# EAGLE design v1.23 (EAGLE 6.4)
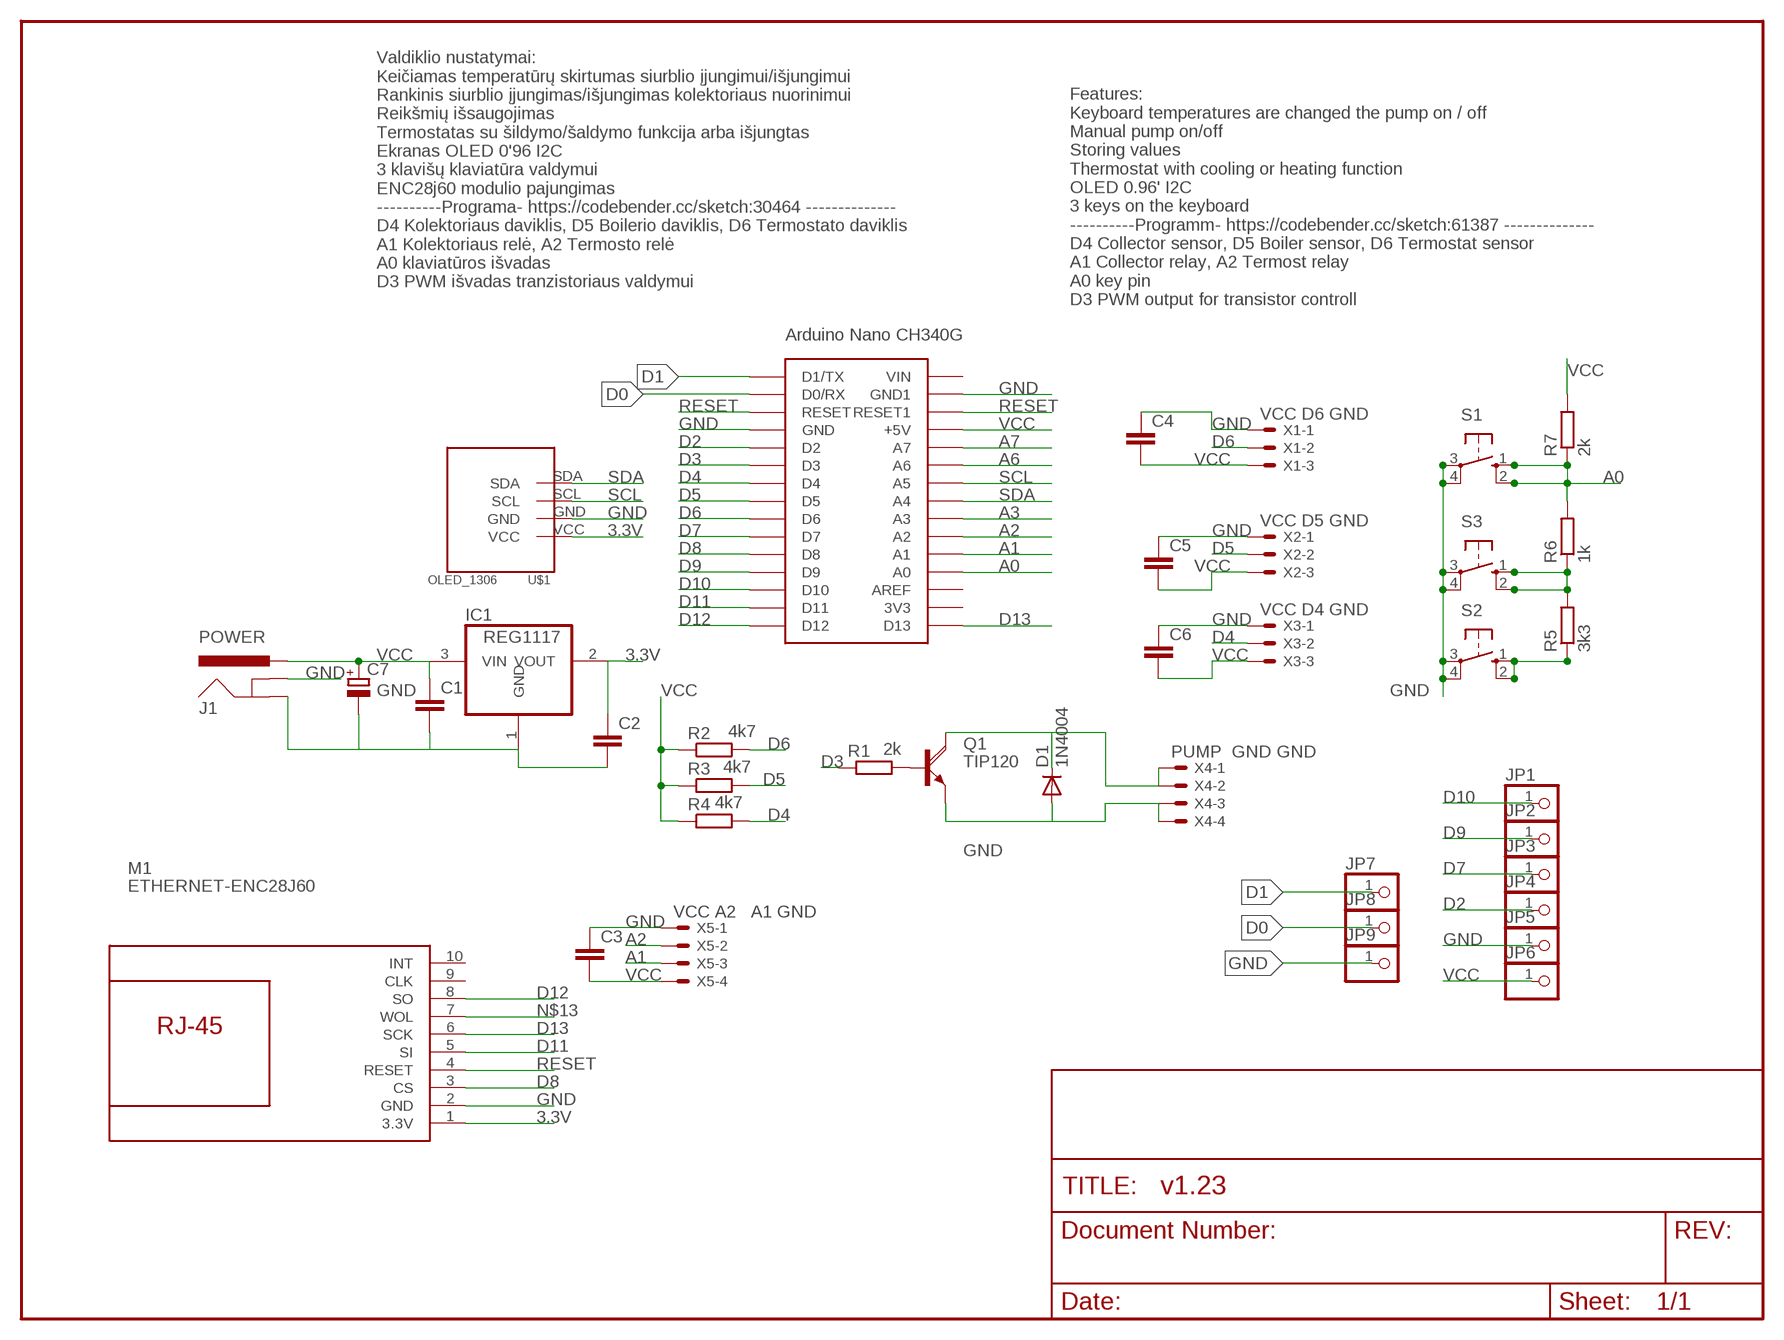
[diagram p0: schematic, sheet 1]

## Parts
ARDUINONANOCH340G  ARDUINONANO  [PDIP-32]
C1  C2,5-3  [C2.5-3]
C2  C2,5-3  [C2.5-3]
C3  C2,5-3  [C2.5-3]
C4  C2,5-3  [C2.5-3]
C5  C2,5-3  [C2.5-3]
C6  C2,5-3  [C2.5-3]
C7  CPOL-EUE2,5-6E  [E2,5-6E]
D1  1N4004  [DO41-10]
IC1  REG1117  [SOT223]
J1  POWER  POWER_JACKPTH_LOCK  [POWER_JACK_PTH_LOCK]
JP1  PINHD-1X1  [1X01]
JP2  PINHD-1X1  [1X01]
JP3  PINHD-1X1  [1X01]
JP4  PINHD-1X1  [1X01]
JP5  PINHD-1X1  [1X01]
JP6  PINHD-1X1  [1X01]
JP7  PINHD-1X1  [1X01]
JP8  PINHD-1X1  [1X01]
JP9  PINHD-1X1  [1X01]
M1  ETHERNET-ENC28J60  [ETHERNET-ENC28J60]
Q1  TIP120  [TO220AH]
R1  2k  R-EU_0207/10  [0207/10]
R2  4k7  R-EU_0207/10  [0207/10]
R3  4k7  R-EU_0207/10  [0207/10]
R4  4k7  R-EU_0207/10  [0207/10]
R5  3k3  R-EU_0207/10  [0207/10]
R6  1k  R-EU_0207/10  [0207/10]
R7  2k  R-EU_0207/10  [0207/10]
S1  10-XX  [B3F-10XX]
S2  10-XX  [B3F-10XX]
S3  10-XX  [B3F-10XX]
U$1  OLED_1306  [OLED_1306]
X1  VCC D6 GND  22-23-2031  [22-23-2031]
X2  VCC D5 GND  22-23-2031  [22-23-2031]
X3  VCC D4 GND  22-23-2031  [22-23-2031]
X4  PUMP GND GND  22-23-2041  [22-23-2041]
X5  VCC A2 A1 GND  22-23-2041  [22-23-2041]

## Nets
3.3V: C2.1 IC1.2(VOUT) M1.1(3.3V) U$1.VCC
A0: ARDUINONANOCH340G.A0 R6.2 R7.1 S1.1(S) S1.2(S1)
A1: ARDUINONANOCH340G.A1 X5.3
A2: ARDUINONANOCH340G.A2 X5.2
A3: ARDUINONANOCH340G.A3
A6: ARDUINONANOCH340G.A6
A7: ARDUINONANOCH340G.A7
D0: ARDUINONANOCH340G.D0/RX JP8.1
D1: ARDUINONANOCH340G.D1/TX JP7.1
D2: ARDUINONANOCH340G.D2 JP4.1
D3: ARDUINONANOCH340G.D3 R1.1
D4: ARDUINONANOCH340G.D4 R4.2 X3.2
D5: ARDUINONANOCH340G.D5 R3.2 X2.2
D6: ARDUINONANOCH340G.D6 R2.2 X1.2
D7: ARDUINONANOCH340G.D7 JP3.1
D8: ARDUINONANOCH340G.D8 M1.3(CS)
D9: ARDUINONANOCH340G.D9 JP2.1
D10: ARDUINONANOCH340G.D10 JP1.1
D11: ARDUINONANOCH340G.D11 M1.5(SI)
D12: ARDUINONANOCH340G.D12 M1.8(SO)
D13: ARDUINONANOCH340G.D13 M1.6(SCK)
GND [vcc]: ARDUINONANOCH340G.GND ARDUINONANOCH340G.GND1 C1.2 C2.2 C3.1 C4.1 C5.1 C6.1 C7.- D1.A IC1.1(GND) J1.GND J1.GNDBREAK JP5.1 JP9.1 M1.2(GND) Q1.E S1.3(P) S1.4(P1) S2.3(P) S2.4(P1) S3.3(P) S3.4(P1) U$1.GND X1.1 X2.1 X3.1 X4.3 X4.4 X5.1
N$1: Q1.B R1.2
N$2: D1.C Q1.C X4.1 X4.2
N$5: R5.1 S2.1(S) S2.2(S1)
N$6: R5.2 R6.1 S3.1(S) S3.2(S1)
N$13: M1.7(WOL)
RESET: ARDUINONANOCH340G.RESET ARDUINONANOCH340G.RESET1 M1.4(RESET)
SCL: ARDUINONANOCH340G.A5 U$1.SCL
SDA: ARDUINONANOCH340G.A4 U$1.SDA
VCC: ARDUINONANOCH340G.+5V C1.1 C3.2 C4.2 C5.2 C6.2 C7.+ IC1.3(VIN) J1.PWR JP6.1 R2.1 R3.1 R4.1 R7.2 X1.3 X2.3 X3.3 X5.4
Unconnected: ARDUINONANOCH340G.3V3 ARDUINONANOCH340G.AREF ARDUINONANOCH340G.VIN M1.9(CLK) M1.10(INT)

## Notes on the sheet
- Valdiklio nustatymai:
  Keičiamas temperatūrų skirtumas siurblio įjungimui/išjungimui
  Rankinis siurblio įjungimas/išjungimas kolektoriaus nuorinimui
  Reikšmių išsaugojimas
  Termostatas su šildymo/šaldymo funkcija arba išjungtas
  Ekranas OLED 0'96 I2C
  3 klavišų klaviatūra valdymui
  ENC28j60 modulio pajungimas
  ----------Programa- https://codebender.cc/sketch:30464 --------------
  D4 Kolektoriaus daviklis, D5 Boilerio daviklis, D6 Termostato daviklis
  A1 Kolektoriaus relė, A2 Termosto relė
  A0 klaviatūros išvadas 
  D3 PWM išvadas tranzistoriaus valdymui
- Features:
  Keyboard temperatures are changed the pump on / off
  Manual pump on/off
  Storing values
  Thermostat with cooling or heating function
  OLED 0.96' I2C
  3 keys on the keyboard
  ----------Programm- https://codebender.cc/sketch:61387 --------------
  D4 Collector sensor, D5 Boiler sensor, D6 Termostat sensor
  A1 Collector relay, A2 Termost relay
  A0 key pin 
  D3 PWM output for transistor controll
- Arduino Nano CH340G

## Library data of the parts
ARDUINONANOCH340G = rocketfarm:ARDUINONANO
C1-C6 = capacitor-wima:C: CAPACITOR
C7 = resistor:CPOL-EU: POLARIZED CAPACITOR, European symbol
D1 = diode:1N4004: DIODE
IC1 = burr-brown:REG1117: 800mA and 1A Low Dropout (LDO) Positive Regulator 1.8V, 2.5V, 2.85V, 3.3V, 5V, and Adj; MPN: REG1117; OC_FARNELL: 1097566; OC_NEWARK: 14P6981
J1 = SparkFun-Connectors:POWER_JACK: Power Jack This is the standard 5.5mm barrel jack for power. The PTH is the most common, proven, reliable, footprint. The Slot footprint only works if the mill layer is transmitted to the PCB fab house so be warned. Spark Fun Electronics SKU : PRT-00119 SMT: CONN-08106 Mating wall wart : TOL-00298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
JP1-JP9 = pinhead:PINHD-1X1: PIN HEADER
M1 = diy-modules:ETHERNET-ENC28J60: Ethernet Module based on ENC28J60 chip
Q1 = transistor-power:TIP120: NPN DARLINGTON TRANSISTOR
R1-R7 = resistor:R-EU_: RESISTOR, European symbol
S1-S3 = switch-omron:10-XX: OMRON SWITCH; MPN: B3F-1000; OC_FARNELL: 176432; OC_NEWARK: 36M3542
U$1 = tft_1.8:OLED_1306
X1-X3 = con-molex:22-23-2031: .100" (2.54mm) Center Header - 3 Pin; MF: MOLEX; MPN: 22-23-2031; OC_FARNELL: 1462950; OC_NEWARK: 30C0862
X4 X5 = con-molex:22-23-2041: .100" (2.54mm) Center Header - 4 Pin; MF: MOLEX; MPN: 22-23-2041; OC_FARNELL: 1462920; OC_NEWARK: 38C0355

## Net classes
0 default: width 0.3 mm
1 vcc: width 0.4 mm
2 gnd: width 0.5 mm

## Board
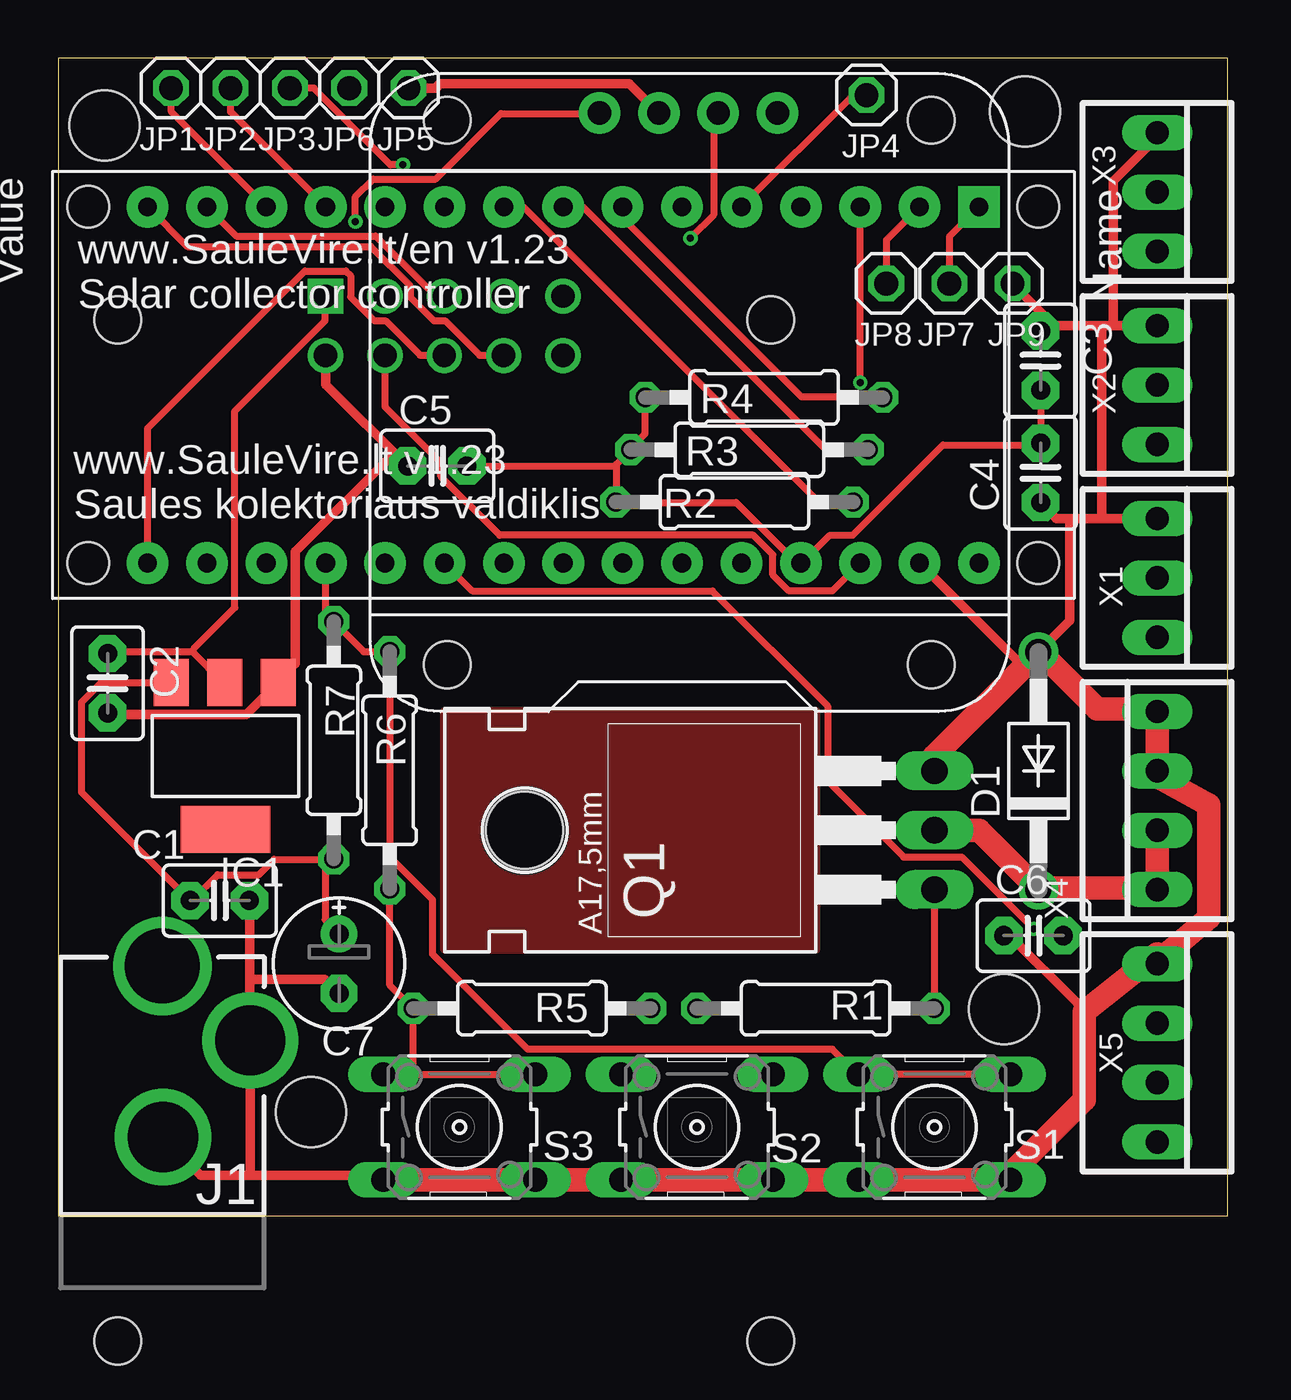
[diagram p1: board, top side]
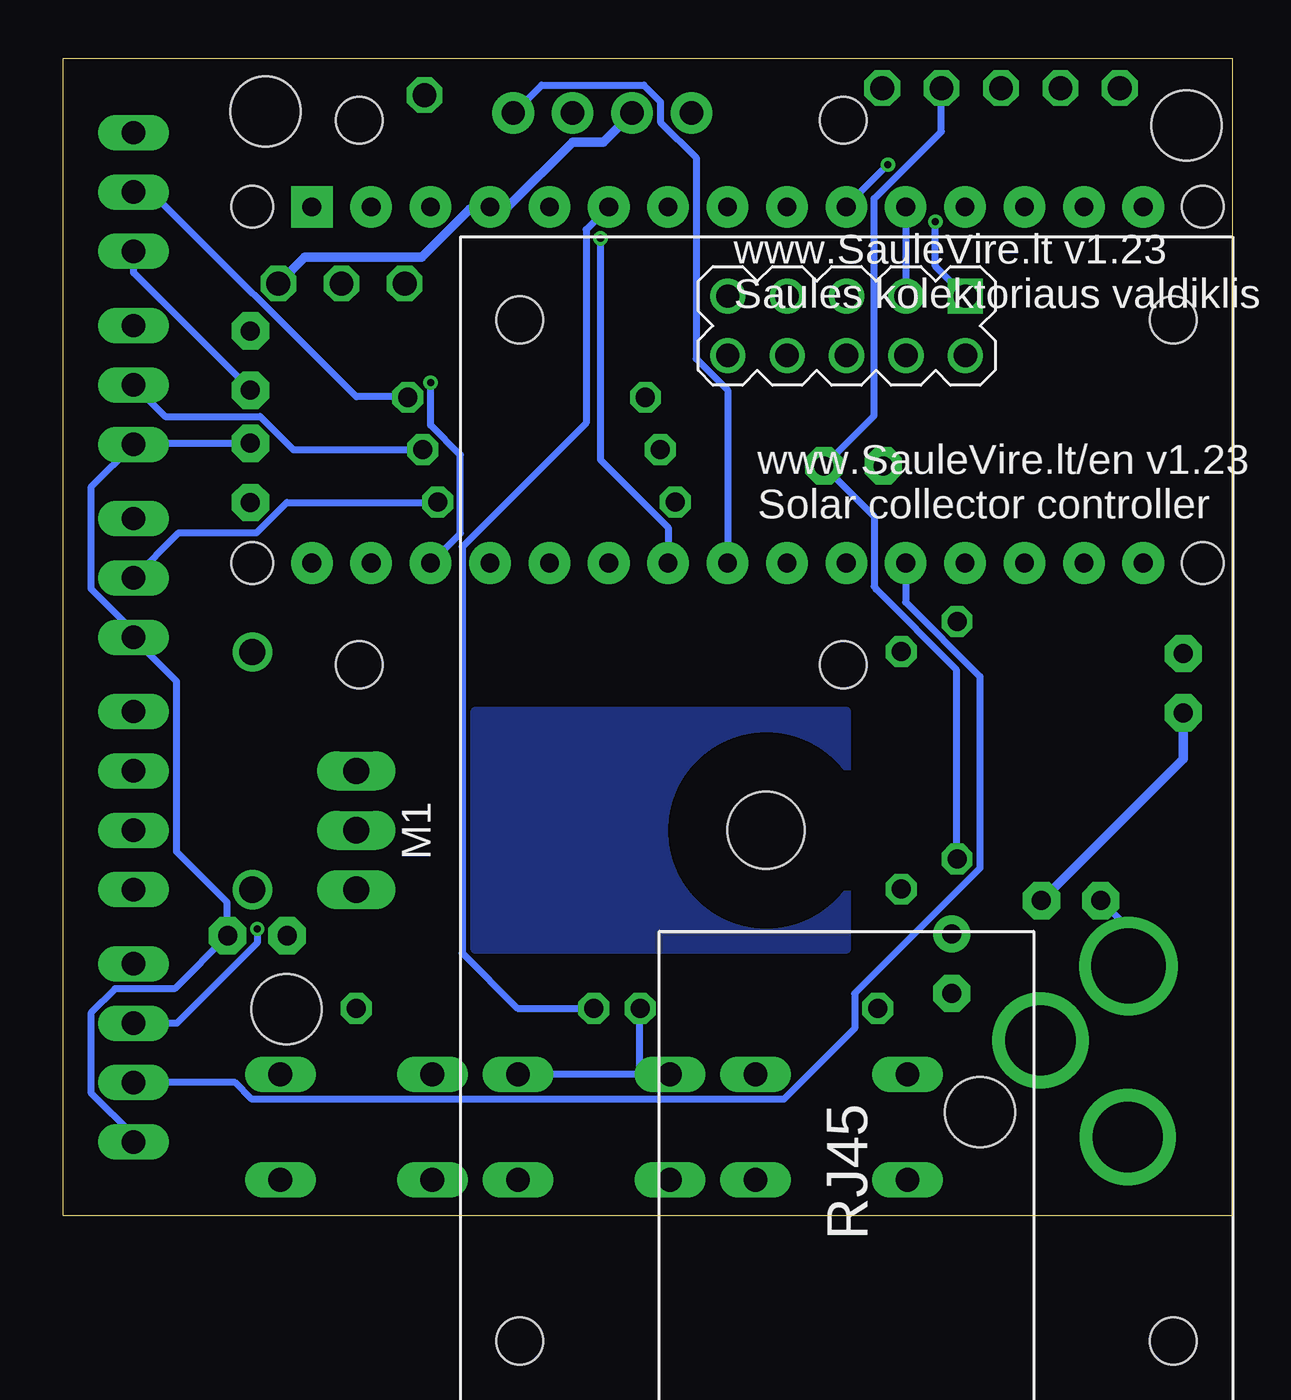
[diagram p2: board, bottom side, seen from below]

Size 50 x 49.51 mm. Coordinates in mm from the lower left corner, seen from the top.
Outline: 0,49.51 0,0 50,0 50,49.51 0,49.51
Copper layers (1*16): Top 0.035mm / dielectric 1.5mm / Bottom 0.035mm
Design rules "ITEADstudio_DRC": minimum track width 6mil, minimum drill 12mil, track to track 6mil, track to pad 6mil, pad to pad 6mil, via to via 6mil, smd to smd 0mil, copper to edge 10mil, drill to drill 10mil, minimum pad ring 10mil, minimum via ring 6mil, stop-mask expansion 2mil, vias tented up to drill 100mil, thermal gap 10mil
Holes 3 mm at 1.97,46.64 10.79,4.43 40.45,8.84 41.34,47.24

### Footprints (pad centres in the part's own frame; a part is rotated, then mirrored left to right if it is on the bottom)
PDIP-32 = drill 0.8 pad 1.778: 3V3 15.24,-35.56; +5V 15.24,-10.16; A0 15.24,-30.48; A1 15.24,-27.94; A2 15.24,-25.4; A3 15.24,-22.86; A4 15.24,-20.32; A5 15.24,-17.78; A6 15.24,-15.24; A7 15.24,-12.7; AREF 15.24,-33.02; D0/RX 0,-5.08; D2 0,-12.7; D3 0,-15.24; D4 0,-17.78; D5 0,-20.32; D6 0,-22.86; D7 0,-25.4; D8 0,-27.94; D9 0,-30.48; D10 0,-33.02; D11 0,-35.56; D12 0,-38.1; D13 15.24,-38.1; GND 0,-10.16; GND1 15.24,-5.08; RESET 0,-7.62; RESET1 15.24,-7.62; VIN 15.24,-2.54 | drill 0.8 pad 1.778 square: D1/TX 0,-2.54 | hole 1.778: 0,0; 0,-40.64; 15.24,-40.64; 15.24,0
C2.5-3 = drill 0.813 pad 1.6 octagon: 1 -1.27,0; 2 1.27,0
E2,5-6E = drill 0.813 pad 1.575: + -1.27,0 | drill 0.813 pad 1.575 octagon: - 1.27,0
DO41-10 = drill 1.118: A 5.08,0; C -5.08,0
SOT223 = smd 1.499 x 2.007: 1 -2.261,-3.15; 2 0.025,-3.15; 3 2.311,-3.15 | smd 3.81 x 2.007: 4 0,3.15
POWER_JACK_PTH_LOCK = drill 2.997 pad 4.115: GND 0.025,6.557; GNDBREAK 3.762,10.7 | drill 3.2 pad 4.115: PWR 0,13.878
1X01 = drill 1.016 octagon: 1 0,0
ETHERNET-ENC28J60 = drill 1 square: 1 22.86,-5.08 | drill 1: 2 20.32,-5.08; 3 22.86,-2.54; 4 20.32,-2.54; 5 22.86,0; 6 20.32,0; 7 22.86,2.54; 8 20.32,2.54; 9 22.86,5.08; 10 20.32,5.08 | hole 2: -21.844,13.97; 21.844,13.97; -21.844,-13.97; 21.844,-13.97
TO220AH = drill 1.118 long: B -2.54,-6.35; C 0,-6.35; E 2.54,-6.35 | hole 3.302: 0,11.176
0207/10 = drill 0.813 octagon: 1 -5.08,0; 2 5.08,0
B3F-10XX = drill 1.016 long: 1 -3.251,2.261; 2 3.251,2.261; 3 -3.251,-2.261; 4 3.251,-2.261
OLED_1306 = drill 1 pad 1.778: GND -0.36,11.63; SCL 2.18,11.63; SDA 4.72,11.63; VCC -2.9,11.63 | hole 2: -9.4,-11.97; 11.3,-11.97; 11.3,11.33; -9.4,11.33
22-23-2031 = drill 1 long: 1 -2.54,0; 2 0,0; 3 2.54,0
22-23-2041 = drill 1 long: 1 -3.81,0; 2 -1.27,0; 3 1.27,0; 4 3.81,0

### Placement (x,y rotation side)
ARDUINONANOCH340G  41.91,43.16 270 top
C1  6.9,13.48 0 top
C2  2.1,22.78 270 top
C3  42,36.58 270 top
C4  42,31.78 90 top
C5  16.2,32.08 0 top
C6  41.7,11.98 0 top
C7  12,10.78 270 top
D1  41.91,19.03 90 top
IC1  7.14,19.66 180 top
J1  4.45,-3.19 0 top
JP1  4.82,48.24 0 top
JP2  7.36,48.24 0 top
JP3  9.89,48.24 0 top
JP4  34.55,47.94 0 top
JP5  14.97,48.24 0 top
JP6  12.44,48.24 0 top
JP7  38.1,39.88 0 top
JP8  35.4,39.88 0 top
JP9  40.8,39.88 0 top
M1  16.5,16.48 90 bottom
Q1  31.11,16.49 90 top
R1  32.38,8.87 0 top
R2  28.91,30.53 0 top
R3  29.55,32.77 0 top
R4  30.18,35.01 0 top
R5  20.25,8.87 180 top
R6  14.16,19.05 90 top
R7  11.78,20.34 270 top
S1  37.47,3.79 0 top
S2  27.3,3.79 0 top
S3  17.14,3.79 0 top
U$1  26.04,35.54 0 top
X1  46.99,27.29 270 top
X2  46.99,35.54 270 top
X3  46.99,43.79 270 top
X4  46.99,17.76 90 top
X5  46.99,6.97 270 top

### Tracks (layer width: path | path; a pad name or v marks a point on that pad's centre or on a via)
3.3V  (via drill 0.3)
  Top 0.3: IC1.2 7.04,22.82 5.71,24.14 | 5.71,24.14 2.18,24.14 C2.1 | M1.1 11.4,39.32 11.4,38.28 7.54,34.42 7.54,26.02 5.79,24.26 5.71,24.14 | v12.7,42.52 12.7,43.59 13.46,44.35 16.13,44.35 18.92,47.15 23.11,47.15 U$1.VCC
  Bottom 0.3: v12.7,42.52 12.7,40.62 M1.1
A0
  Top 0.3: S1.2 S1.1 34.09,6.13 33.1,7.12 20.07,7.12 16,11.18 16,13.52 14.2,15.32 14.2,23.98 R6.2 14.15,24.14 13.06,24.14 11.89,25.3 R7.1 11.71,25.56 11.43,25.84 ARDUINONANOCH340G.A0
A1
  Bottom 0.3: X5.3 42.65,5.7 41.94,4.98 19.18,4.98 16.15,8.01 16.15,9.51 10.79,14.86 10.79,23.07 13.97,26.24 ARDUINONANOCH340G.A1
A2  (via drill 0.3)
  Top 0.3: v41.71,12.27 38.63,15.35 36.14,15.35 32.89,18.6 32.89,21.8 27.96,26.73 17.7,26.73 ARDUINONANOCH340G.A2
  Bottom 0.3: X5.2 45.14,8.24 41.71,11.66 v41.71,12.27
D0
  Top 0.3: ARDUINONANOCH340G.D0/RX 35.41,41.74 JP8.1
D1
  Top 0.3: JP7.1 38.1,41.89 ARDUINONANOCH340G.D1/TX
D2
  Top 0.3: ARDUINONANOCH340G.D2 33.98,47.93 JP4.1
D3
  Bottom 0.3: R1.1 30.58,8.87 32.94,11.23 32.94,28.61 27.64,33.91 27.64,42.2 ARDUINONANOCH340G.D3
D4
  Top 0.3: ARDUINONANOCH340G.D4 24.13,42.68 31.77,35.03 35.26,35.03 R4.2
  Bottom 0.3: X3.2 46.23,43.79 37.47,35.03 35.28,35.03 R4.2
D5
  Top 0.3: ARDUINONANOCH340G.D5 22.43,43.16 32.82,32.77 R3.2
  Bottom 0.3: X2.2 45.64,34.19 41.58,34.19 40.16,32.77 34.65,32.77 R3.2
D6
  Top 0.3: ARDUINONANOCH340G.D6 19.89,43.16 32.51,30.54 R2.2
  Bottom 0.3: X1.2 45.06,29.21 41.73,29.21 40.44,30.51 34.01,30.51 R2.2
D7  (via drill 0.3)
  Top 0.3: JP3.1 10.92,48.24 14.2,44.96 v14.73,44.96
  Bottom 0.3: v14.73,44.96 16.51,43.18 ARDUINONANOCH340G.D7
D8
  Bottom 0.3: ARDUINONANOCH340G.D8 M1.3
D9
  Top 0.3: ARDUINONANOCH340G.D9 7.37,47.22 JP2.1
D10
  Top 0.3: ARDUINONANOCH340G.D10 4.83,47.22 JP1.1
D11
  Top 0.3: ARDUINONANOCH340G.D11 7.59,41.91 13.56,41.91 16.13,39.35 16.48,39.35 M1.5
D12
  Top 0.3: ARDUINONANOCH340G.D12 5.51,41.46 13.36,41.46 15.04,39.78 15.04,39.3 16.05,38.28 16.54,38.28 18.01,36.81 19.02,36.81 M1.8
D13
  Top 0.3: ARDUINONANOCH340G.D13 3.81,33.69 10.54,40.42 12.29,40.42 12.5,40.21 12.5,39.3 13.51,38.28 13.99,38.28 15.47,36.81 16.48,36.81 M1.6
GND
  Top 0.4: 46.99,11.21 X5.1 47.09,10.95 | 40.92,2.01 S1.4 | D1.A 41.26,23.46 40.95,23.8 ARDUINONANOCH340G.GND1 | 46.81,21.67 X4.4 | 42.09,24.01 D1.A | 42.22,24.16 D1.A | 47.09,18.73 47.09,18.85 X4.3 | 8.2,1.73 6.1,1.73 J1.GND | 8.2,1.73 13.41,1.73 S3.3 | 8.2,1.73 8.2,7.3 J1.GNDBREAK 8.18,7.7 8.18,10.12 | JP5.1 16.13,48.24 16.31,48.42 24.41,48.42 25.65,47.17 U$1.GND | 44.63,38.08 42.24,38.08 42.01,37.85 C3.1 42.42,38.26 40.82,39.86 JP9.1 | 44.63,38.08 45.11,38.08 | 45.11,38.08 X2.1 | X3.1 46.99,46.13 45.11,44.25 45.11,38.08 | M1.2 11.43,36.78 11.43,35.56 14.91,32.09 C5.1 14.22,32.49 10.13,28.4 10.13,23.63 9.5,22.99 IC1.1 9.4,22.82 8.03,21.44 2.16,21.44 2.11,21.49 C2.2 | 43.26,29.82 42.67,29.82 42.01,30.48 C4.1 | 43.26,29.82 44.63,29.82 | 44.63,29.82 X1.1 | 8.18,10.12 8.18,13.47 C1.2 | C6.1 40.69,11.97 43.56,9.1 43.87,8.72 | 43.26,29.82 43.26,25.46 D1.A | 44.63,29.82 44.63,38.08 | 8.18,10.12 11.38,10.12 C7.-
  Top 1: S3.3 S3.4 S2.3 S2.4 S1.3 S1.4 | 46.99,11.21 43.87,8.72 43.87,4.96 40.92,2.01 | X4.4 X4.3 | Q1.E 37.47,19.66 41.26,23.46 | 46.81,21.67 44.42,21.67 42.09,24.01 | 47.09,18.73 49.2,17.58 49.2,12.73 47.09,10.95
  Bottom 0.4: U$1.GND 25.68,47.15 26.9,45.93 28.22,45.93 30.99,43.16 ARDUINONANOCH340G.GND 31.93,43.06 32.61,43.06 34.67,41 39.67,41 JP9.1 | C2.2 2.11,21.49 2.11,19.54 8.15,13.49 C1.2
N$1
  Top 0.3: Q1.B R1.2
N$2
  Top 0.3: 46.86,14.03 X4.1 | 42.04,14.03 D1.C
  Top 1: X4.2 X4.1 | Q1.C 39.37,16.49 D1.C | 42.04,14.03 46.86,14.03
N$3
  pour Bottom: 16.51,21.57 32.38,21.57 32.38,11.41 16.51,11.41
N$4
  pour Top: 16.51,21.57 32.38,21.57 32.38,11.41 16.51,11.41
N$5
  Bottom 0.3: S2.1 S2.2 | 24.13,6.18 S2.1 | R5.1 25.35,8.87 25.35,6.18 S2.1
N$6
  Top 0.3: S3.2 S3.1 15.16,6.18 15.16,8.74 R5.2 14.17,9.86 14.17,13.95 R6.1
RESET  (via drill 0.3)
  Top 0.3: ARDUINONANOCH340G.RESET1 33.1,26.73 31.24,26.73 30.56,27.41 30.56,28.28 29.72,29.11 18.87,29.11 16.36,31.63 16.36,32.21 13.97,34.6 13.97,36.78 M1.4 | v34.29,35.64 ARDUINONANOCH340G.RESET
  Bottom 0.3: v34.29,35.64 34.29,33.81 33.02,32.54 33.02,29.19 ARDUINONANOCH340G.RESET1
SCL  (via drill 0.3)
  Top 0.3: v27.03,41.81 28.02,42.8 28.02,46.97 28.19,47.15 U$1.SCL
  Bottom 0.3: ARDUINONANOCH340G.A5 24.13,29.44 27.03,32.34 v27.03,41.81
SDA
  Bottom 0.3: ARDUINONANOCH340G.A4 21.59,35.31 22.94,36.66 22.94,45.27 24.46,46.79 24.46,47.66 25.17,48.37 29.54,48.37 30.73,47.17 U$1.SDA
VCC
  Top 0.3: C3.2 42.01,35.29 42.01,33.05 C4.2 41.86,32.97 37.82,32.97 33.96,29.11 32.99,29.11 31.88,28 ARDUINONANOCH340G.+5V 31.57,27.92 28.98,30.51 24,30.51 R2.1 23.85,30.54 23.85,32.06 | IC1.3 1.83,22.82 0.99,21.98 0.99,18.12 5.61,13.49 C1.1 5.77,13.54 6.81,14.59 8.56,14.59 9.22,15.25 11.76,15.25 R7.2 11.4,15.12 11.4,12.66 C7.+ | 23.85,32.06 23.85,32.14 24.46,32.75 R3.1 24.54,32.9 25.09,33.46 R4.1 | 23.85,32.06 17.48,32.06 C5.2
  Bottom 0.3: 46.86,24.82 X1.3 | 4.45,10.7 J1.PWR 4.52,10.83 4.52,12.38 5.61,13.47 C1.1 | X5.4 46.99,3.43 48.82,5.26 48.82,8.67 47.78,9.71 45.24,9.71 C6.2 43,12.12 43,13.42 45.16,15.58 45.16,22.87 46.91,24.62 X1.3 | X1.3 46.94,24.95 48.82,26.83 48.82,31.17 X2.3 46.86,33.02 42.01,33.02 C4.2 | X3.3 46.99,40.34 42.01,35.36 42.01,35.31 C3.2 | JP6.1 12.45,46.39 15.32,43.52 15.32,34.22 17.45,32.09 C5.2 17.37,31.96 15.32,29.9 15.32,26.93 15.24,26.8 11.81,23.37 11.81,15.42 R7.2 11.79,15.27

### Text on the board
tPlace: www.SauleVire.lt/en v1.23 / Solar collector controller | www.SauleVire.lt v1.23 / Saules kolektoriaus valdiklis
bPlace: www.SauleVire.lt v1.23 / Saules kolektoriaus valdiklis | www.SauleVire.lt/en v1.23 / Solar collector controller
